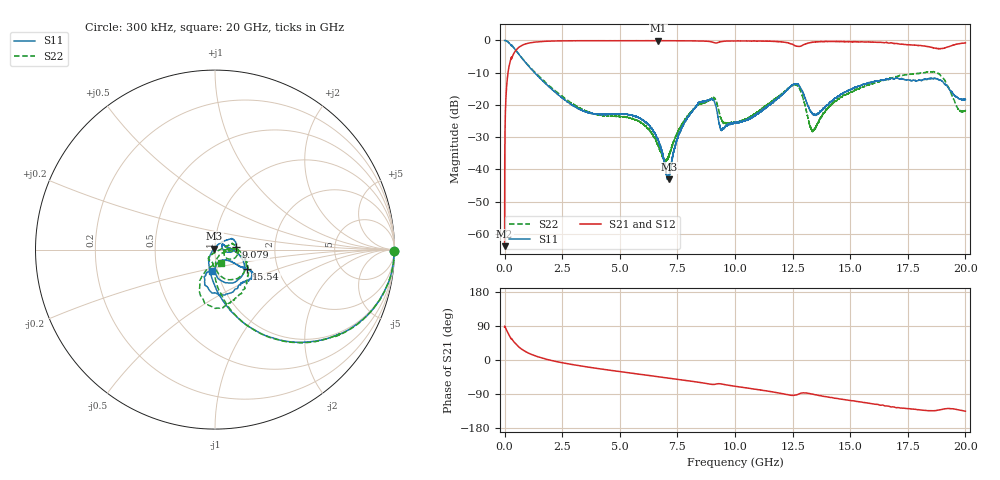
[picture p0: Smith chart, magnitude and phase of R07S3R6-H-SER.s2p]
!{R07S3R6}
!Johanson Technology Inc.
!www.johansontechnology.com
!Test Board Conditions:
!Substrate Type  RO4350B
!Substrate Thickness  10 mil
!Substrate Dk  3.66
!TL Type: GCPW
!TL Trace Width  21 mil
!TL Gap  20 mil
!Electrode orientation  Horizontal
!DUT TOPOLOGY	SERIES
!Mounting Pad LxW  16x21 mil
! Created Sat Feb  6 11:31:41 2021
# hz S ma R 50
! 2 Port Network Data from SP1.SP block
! freq  magS11  angS11  magS21  angS21  magS12  angS12  magS22  angS22
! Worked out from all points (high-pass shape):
!   20001 points, 300 kHz to 20 GHz, reference 50 ohm
!   highest |S21| = -0.06 dB at 6.677 GHz (marker M1); lowest = -63.9 dB at 300 kHz (marker M2)
!   |S21| within 3 dB of the highest: 488.5 MHz to end of sweep
!   lowest |S11| = -43.1 dB at 7.132 GHz (marker M3), VSWR 1.01, Z = 49.6 + j0.585 ohm
!   |S11| at or under -10 dB: 1.301 GHz to end of sweep
!   |S22| runs from -37.7 to 0.0 dB; largest |S21 - S12| = 0.013
!   S11 on the Smith chart (normalised r, x): 300 kHz: open; 9.079 GHz: 1.27, +0.03; 15.54 GHz: 1.39, -0.32; 20 GHz: 0.94, -0.23
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300000  0.9997 -0.5  0.0006409 86.4  0.0006585 94.0  1 -0.5
1.183e8  0.965 -15.5  0.2563 74.7  0.2563 74.7  0.9661 -15.5
3.673e8  0.7959 -38.6  0.5951 50.8  0.5961 50.8  0.7969 -38.6
1.2323e9  0.3362 -76.9  0.9346 13.1  0.934 13.1  0.344 -75.6
3.3343e9  0.08305 -114.5  0.9906 -15.9  0.9906 -15.9  0.08672 -96.1
5.7313e9  0.06544 -122.0  0.9916 -36.5  0.9911 -36.5  0.05786 -128.6
6.6673e9  0.0287 -137.6  0.9923 -44.2  0.9917 -44.2  0.02392 -114.1
6.6773e9  0.02765 -138.7  0.9933 -44.3  0.9919 -44.3  0.02307 -113.6
7.1323e9  0.007032 123.0  0.9918 -47.9  0.9916 -48.0  0.01637 -24.0
7.4843e9  0.02877 60.4  0.9911 -50.9  0.9899 -50.9  0.03605 6.7
7.8833e9  0.05801 47.2  0.987 -54.2  0.9872 -54.3  0.06233 14.5
8.4873e9  0.1102 33.7  0.9803 -59.4  0.9802 -59.4  0.1024 19.7
9.0793e9  0.1181 6.1  0.9282 -64.6  0.9269 -64.6  0.1289 -9.6
9.4173e9  0.0405 14.0  0.9609 -63.4  0.9591 -63.3  0.05962 -29.9
1.00003e10  0.05271 33.7  0.9842 -69.3  0.9835 -69.4  0.05248 -4.9
1.26043e10  0.2115 -48.5  0.8299 -92.8  0.8296 -93.0  0.2068 -43.4
1.33343e10  0.07506 -77.0  0.9365 -89.7  0.9356 -89.8  0.0402 -55.3
1.42713e10  0.1187 -35.7  0.9633 -100.2  0.9642 -100.1  0.1087 -5.6
1.55433e10  0.2078 -31.8  0.9556 -111.7  0.9525 -111.4  0.1913 -22.1
1.66673e10  0.2477 -33.4  0.9092 -121.8  0.9139 -122.2  0.2555 -46.1
1.87873e10  0.2539 -84.8  0.7512 -132.6  0.7484 -132.6  0.31 -97.4
2e10  0.1212 -97.2  0.9171 -135.2  0.9136 -135.1  0.08204 -63.2
